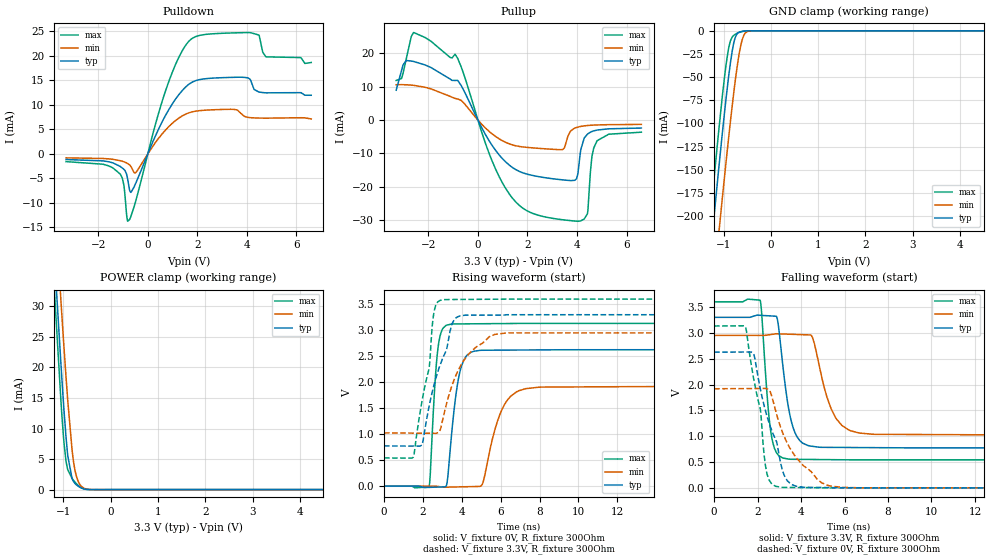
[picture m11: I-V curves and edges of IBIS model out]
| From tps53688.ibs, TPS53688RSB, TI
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|   out Model
[Model]   out
Model_type   3-state
Polarity   Non-Inverting
Vmeas = 1.65
Vref = 0
Cref = 2pF
Rref = 100000
|   typ   min   max
C_comp   1.878pF   1.852pF   1.904pF
[Voltage Range]   3.3   2.95   3.6
|Junction Temperature
[Temperature Range]   25   125   -40
[Pullup Reference]   3.3   2.95   3.6
[Pulldown Reference]   0   0   0
[Power Clamp Reference]   3.3   2.95   3.6
[GND Clamp Reference]   0   0   0
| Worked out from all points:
|   slope of the pulldown table from 0 to 0.495 V, typ, clamps not added: 87.2 ohm
|   slope of the pullup table from 0 to 0.495 V, typ, clamps not added: 73.6 ohm
|   GND clamp passes 1 mA (typ) near -0.64 V on its own axis
|   POWER clamp passes 1 mA (typ) near -0.75 V on its own axis
|   falling waveform, V_fixture 3.3V, R_fixture 300Ohm: 20-80 % time 506ps typ, 793ps min, 338ps max; typ from 3.3 V to 0.774 V
|   rising waveform, V_fixture 0V, R_fixture 300Ohm: 20-80 % time 484ps typ, 871ps min, 301ps max; typ from 0 V to 2.63 V
|   rising waveform, V_fixture 3.3V, R_fixture 300Ohm: 20-80 % time 1.11ns typ, 1.32ns min, 717ps max; typ from 0.774 V to 3.3 V
|   falling waveform, V_fixture 0V, R_fixture 300Ohm: 20-80 % time 999ps typ, 1.45ns min, 641ps max; typ from 2.63 V to 0 V
[Pulldown]
|   Voltage   I(typ)   I(min)   I(max)
-3.3V     -1.14mA    -802.1uA   -1.57mA
-1.122V   -2.526mA   -1.372mA   -4.066mA
-973.5mV  -3.112mA   -1.585mA   -6.194mA
-815.1mV  -5.079mA   -1.949mA   -13.74mA
-676.5mV  -7.825mA   -2.595mA   -12.65mA
-478.5mV  -5.867mA   -3.748mA   -9.444mA
709.5mV   7.793mA    4.84mA     12.75mA
1.68V     14.28mA    8.413mA    23.08mA
4.155V    14.98mA    7.386mA    24.7mA
4.491V    12.63mA    7.31mA     24.18mA
4.769V    12.46mA    7.292mA    19.79mA
6.6V      11.96mA    7.123mA    18.64mA
[GND Clamp]
|   Voltage   I(typ)   I(min)   I(max)
-3.3V     -1.399A    -1.449A    -1.376A
-1.29V    -248.6mA   -318.7mA   -208.2mA
-1.28V    -243.3mA   -313.4mA   -202.7mA
-1.201V   -200.8mA   -271.3mA   -159.8mA
-1.102V   -149.1mA   -219.7mA   -108.2mA
-1.033V   -114.2mA   -184.3mA   -74.17mA
-904.2mV  -54.41mA   -121.1mA   -22.17mA
-785.4mV  -13.54mA   -67.43mA   -4.957mA
-666.6mV  -1.405mA   -23.95mA   -1.657mA
-567.6mV  -317.4uA   -4.575mA   -424.2uA
-419.1mV  -8.647uA   -102.1uA   -3.992uA
6.6V      0A         0A         0A
[Pullup]
|   Voltage   I(typ)   I(min)   I(max)
-3.3V     8.974mA    10.62mA    11.89mA
-3.023V   16.6mA     10.63mA    14.07mA
-2.607V   17.61mA    10.44mA    26.26mA
-924mV    11.89mA    6.508mA    19.79mA
1.036V    -11.96mA   -6.393mA   -19.5mA
2.788V    -17.41mA   -8.678mA   -29.23mA
3.986V    -17.63mA   -2.214mA   -30.39mA
4.293V    -5.37mA    -1.746mA   -29.72mA
4.432V    -4.18mA    -1.635mA   -27.67mA
4.61V     -3.433mA   -1.541mA   -10.72mA
4.808V    -3.016mA   -1.473mA   -6.279mA
6.6V      -2.401mA   -1.309mA   -3.646mA
[POWER Clamp]
|   Voltage   I(typ)   I(min)   I(max)
-3.3V     348.7mA    341.6mA    365mA
-1.201V   39.85mA    50.03mA    34.33mA
-1.053V   20.95mA    31.28mA    14.88mA
-983.4mV  12.79mA    23.06mA    7.515mA
-943.8mV  8.743mA    18.61mA    4.719mA
-904.2mV  5.478mA    14.45mA    3.222mA
-815.1mV  1.834mA    6.565mA    1.849mA
-765.6mV  1.137mA    3.708mA    1.356mA
-696.3mV  622uA      1.578mA    774.5uA
-607.2mV  228.6uA    465.4uA    255.1uA
-280.5mV  54.03nA    731.6nA    0A
6.6V      0A         0A         0A
[Ramp]
R_load = 300
|   typ   min   max
dV/dt_r   1.57537/4.82298e-10   1.15041/8.69044e-10   1.87914/3.00258e-10
dV/dt_f   1.51558/5.05157e-10   1.1552/7.84897e-10   1.83479/3.37285e-10
[Falling Waveform]
V_fixture = 3.3V
V_fixture_min = 2.95V
V_fixture_max = 3.6V
R_fixture = 300Ohm
C_fixture = 0F
|   Time   V(typ)   V(min)   V(max)
0s        3.3V       2.95V      3.6V
2.118ns   3.339V     2.95V      3.633V
2.478ns   3.33V      2.959V     1.593V
2.654ns   3.326V     2.97V      971.7mV
2.933ns   3.213V     2.981V     644.2mV
3.479ns   1.428V     2.973V     554.1mV
4.475ns   806.7mV    2.95V      549.3mV
5.623ns   782.7mV    1.337V     544.8mV
7.29ns    778.4mV    1.037V     542.1mV
100ns     774mV      1.025V     542mV
[Rising Waveform]
V_fixture = 0V
V_fixture_min = 0V
V_fixture_max = 0V
R_fixture = 300Ohm
C_fixture = 0F
|   Time   V(typ)   V(min)   V(max)
0s        -128.3nV   -410.3nV   -281.3nV
2.312ns   -24.58mV   294.2uV    -15.42mV
2.79ns    -18.1mV    -7.455mV   2.687V
3.223ns   24.27mV    -20.31mV   3.098V
3.479ns   998.3mV    -18.18mV   3.121V
4.293ns   2.529V     -11.39mV   3.124V
5.063ns   2.616V     40.13mV    3.126V
6.373ns   2.619V     1.668V     3.13V
7.975ns   2.622V     1.905V     3.132V
100ns     2.626V     1.917V     3.132V
[Rising Waveform]
V_fixture = 3.3V
V_fixture_min = 2.95V
V_fixture_max = 3.6V
R_fixture = 300Ohm
C_fixture = 0F
|   Time   V(typ)   V(min)   V(max)
0s        774mV      1.025V     542mV
1.52ns    770.7mV    1.02V      560.3mV
1.946ns   787.9mV    1.019V     1.612V
2.328ns   1.547V     1.018V     2.285V
2.579ns   1.953V     1.017V     3.362V
3.08ns    2.51V      1.374V     3.591V
3.732ns   3.248V     2.159V     3.593V
4.563ns   3.292V     2.621V     3.595V
6.334ns   3.3V       2.95V      3.6V
100ns     3.3V       2.95V      3.6V
[Falling Waveform]
|Gnd
V_fixture = 0V
V_fixture_min = 0V
V_fixture_max = 0V
R_fixture = 300Ohm
C_fixture = 0F
|   Time   V(typ)   V(min)   V(max)
0s        2.626V     1.917V     3.132V
1.446ns   2.629V     1.921V     3.112V
1.842ns   2.564V     1.922V     2.069V
2.129ns   1.912V     1.923V     1.518V
2.423ns   1.404V     1.918V     295.3mV
3.119ns   382.4mV    1.108V     10.14mV
3.547ns   68.42mV    731.3mV    7.361mV
4.732ns   7.606mV    173.2mV    2.516mV
5.921ns   3.394mV    8.889mV    54.26uV
100ns     -130.6nV   -712.2nV   -163.2nV
